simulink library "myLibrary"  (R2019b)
settings: Solver=VariableStepAuto  StartTime=0.0  StopTime=10.0  RelTol=1e-3
undefined symbols (not defined in the file or in its folder): batt_delay, Calculation, cap_1ph, cap_3ph, Complex, Current, Dynamic, EV, ev_charger, EV_ID, ev_num, gcbh, Iabc, Load, max_charge_1ph, max_charge_3ph, max_disch_1ph, max_disch_3ph, MV_LV_transf, myLibrary, phase, Phase, Phasor, rated_1ph, rated_3ph, Single, SoC_init, SPDL, sps_rtmsupport, Tr_capacity, Tstep, Vabc, Vnom, yes
libraries: powerlib x163, $bdroot x13, spsVIMeasurementModel x3, simulink x2, powerlib_meascontrol x1
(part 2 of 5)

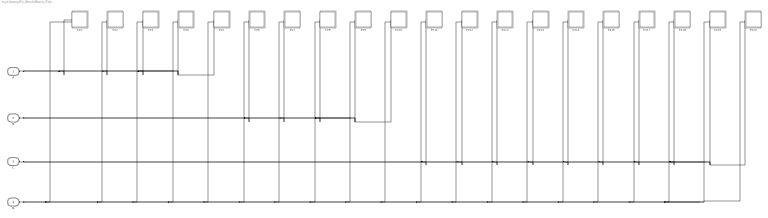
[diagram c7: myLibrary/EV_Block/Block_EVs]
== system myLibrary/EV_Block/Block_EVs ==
  EV1 : Subsystem  mask(Single-Phase Dynamic Load){Load_Profile=EV(1), Phase=1}
      mask prompts: Phase "Phase [A=1, B=2, C=3]"
      mask help: Single Phase Dynamic Load. The Load Profile is given by an external file.
  EV10 : Subsystem  mask(Single-Phase Dynamic Load){Load_Profile=EV(10), Phase=2}
      mask prompts: Phase "Phase [A=1, B=2, C=3]"
      mask help: Single Phase Dynamic Load. The Load Profile is given by an external file.
  EV11 : Subsystem  mask(Single-Phase Dynamic Load){Load_Profile=EV(11), Phase=3}
      mask prompts: Phase "Phase [A=1, B=2, C=3]"
      mask help: Single Phase Dynamic Load. The Load Profile is given by an external file.
  EV12 : Subsystem  mask(Single-Phase Dynamic Load){Load_Profile=EV(12), Phase=3}
      mask prompts: Phase "Phase [A=1, B=2, C=3]"
      mask help: Single Phase Dynamic Load. The Load Profile is given by an external file.
  EV13 : Subsystem  mask(Single-Phase Dynamic Load){Load_Profile=EV(13), Phase=3}
      mask prompts: Phase "Phase [A=1, B=2, C=3]"
      mask help: Single Phase Dynamic Load. The Load Profile is given by an external file.
  EV14 : Subsystem  mask(Single-Phase Dynamic Load){Load_Profile=EV(14), Phase=3}
      mask prompts: Phase "Phase [A=1, B=2, C=3]"
      mask help: Single Phase Dynamic Load. The Load Profile is given by an external file.
  EV15 : Subsystem  mask(Single-Phase Dynamic Load){Load_Profile=EV(15), Phase=3}
      mask prompts: Phase "Phase [A=1, B=2, C=3]"
      mask help: Single Phase Dynamic Load. The Load Profile is given by an external file.
  EV16 : Subsystem  mask(Single-Phase Dynamic Load){Load_Profile=EV(16), Phase=3}
      mask prompts: Phase "Phase [A=1, B=2, C=3]"
      mask help: Single Phase Dynamic Load. The Load Profile is given by an external file.
  EV17 : Subsystem  mask(Single-Phase Dynamic Load){Load_Profile=EV(17), Phase=3}
      mask prompts: Phase "Phase [A=1, B=2, C=3]"
      mask help: Single Phase Dynamic Load. The Load Profile is given by an external file.
  EV18 : Subsystem  mask(Single-Phase Dynamic Load){Load_Profile=EV(18), Phase=3}
      mask prompts: Phase "Phase [A=1, B=2, C=3]"
      mask help: Single Phase Dynamic Load. The Load Profile is given by an external file.
  EV19 : Subsystem  mask(Single-Phase Dynamic Load){Load_Profile=EV(19), Phase=3}
      mask prompts: Phase "Phase [A=1, B=2, C=3]"
      mask help: Single Phase Dynamic Load. The Load Profile is given by an external file.
  EV2 : Subsystem  mask(Single-Phase Dynamic Load){Load_Profile=EV(2), Phase=1}
      mask prompts: Phase "Phase [A=1, B=2, C=3]"
      mask help: Single Phase Dynamic Load. The Load Profile is given by an external file.
  EV20 : Subsystem  mask(Single-Phase Dynamic Load){Load_Profile=EV(20), Phase=3}
      mask prompts: Phase "Phase [A=1, B=2, C=3]"
      mask help: Single Phase Dynamic Load. The Load Profile is given by an external file.
  EV3 : Subsystem  mask(Single-Phase Dynamic Load){Load_Profile=EV(3), Phase=1}
      mask prompts: Phase "Phase [A=1, B=2, C=3]"
      mask help: Single Phase Dynamic Load. The Load Profile is given by an external file.
  EV4 : Subsystem  mask(Single-Phase Dynamic Load){Load_Profile=EV(4), Phase=1}
      mask prompts: Phase "Phase [A=1, B=2, C=3]"
      mask help: Single Phase Dynamic Load. The Load Profile is given by an external file.
  EV5 : Subsystem  mask(Single-Phase Dynamic Load){Load_Profile=EV(5), Phase=1}
      mask prompts: Phase "Phase [A=1, B=2, C=3]"
      mask help: Single Phase Dynamic Load. The Load Profile is given by an external file.
  EV6 : Subsystem  mask(Single-Phase Dynamic Load){Load_Profile=EV(6), Phase=2}
      mask prompts: Phase "Phase [A=1, B=2, C=3]"
      mask help: Single Phase Dynamic Load. The Load Profile is given by an external file.
  EV7 : Subsystem  mask(Single-Phase Dynamic Load){Load_Profile=EV(7), Phase=2}
      mask prompts: Phase "Phase [A=1, B=2, C=3]"
      mask help: Single Phase Dynamic Load. The Load Profile is given by an external file.
  EV8 : Subsystem  mask(Single-Phase Dynamic Load){Load_Profile=EV(8), Phase=2}
      mask prompts: Phase "Phase [A=1, B=2, C=3]"
      mask help: Single Phase Dynamic Load. The Load Profile is given by an external file.
  EV9 : Subsystem  mask(Single-Phase Dynamic Load){Load_Profile=EV(9), Phase=2}
      mask prompts: Phase "Phase [A=1, B=2, C=3]"
      mask help: Single Phase Dynamic Load. The Load Profile is given by an external file.
  A : PMIOPort  Tag=PMCPort  Side=Left
  B : PMIOPort  Tag=PMCPort  Port=2  Side=Left
  C : PMIOPort  Tag=PMCPort  Port=3  Side=Left
  N : PMIOPort  Tag=PMCPort  Port=4  Side=Left
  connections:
  N/RConn1 -- EV1/LConn2 -- EV2/LConn2 -- EV3/LConn2 -- EV4/LConn2 -- EV5/LConn2 -- EV6/LConn2 -- EV7/LConn2 -- EV8/LConn2 -- EV9/LConn2 -- EV10/LConn2 -- EV11/LConn2 -- EV12/LConn2 -- EV13/LConn2 -- EV14/LConn2 -- EV15/LConn2 -- EV16/LConn2 -- EV17/LConn2 -- EV18/LConn2 -- EV20/LConn2 -- EV19/LConn2
  A/RConn1 -- EV1/LConn1 -- EV2/LConn1 -- EV3/LConn1 -- EV5/LConn1 -- EV4/LConn1
  B/RConn1 -- EV6/LConn1 -- EV7/LConn1 -- EV8/LConn1 -- EV10/LConn1 -- EV9/LConn1
  C/RConn1 -- EV11/LConn1 -- EV12/LConn1 -- EV13/LConn1 -- EV14/LConn1 -- EV15/LConn1 -- EV16/LConn1 -- EV17/LConn1 -- EV18/LConn1 -- EV20/LConn1 -- EV19/LConn1

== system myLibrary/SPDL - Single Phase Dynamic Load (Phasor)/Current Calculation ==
  Vp : Inport
  Demux : Demux  Outputs=2
  Divide : Product  Inputs=*/
  From Workspace : FromWorkspace  VariableName=Load_Profile  SampleTime=0  OutputAfterFinalValue=Holding final value
  Gain : Gain  Gain=2
  Math Function : Math  Operator=conj
  Real-Imag to Complex : RealImagToComplex
  Isignal : Outport  VectorParamsAs1DForOutWhenUnconnected=off
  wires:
  From Workspace/1 -> Demux/1
  Real-Imag to Complex/1 -> Gain/1
  Vp/1 -> Divide/2
  Gain/1 -> Divide/1
  Divide/1 -> Math Function/1
  Math Function/1 -> Isignal/1
  Demux/1 -> Real-Imag to Complex/1
  Demux/2 -> Real-Imag to Complex/2

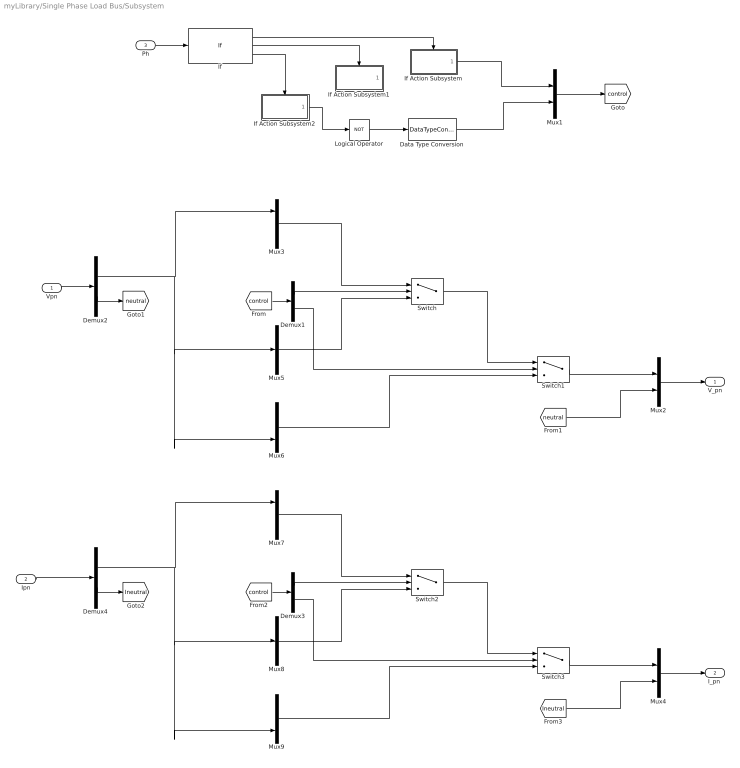
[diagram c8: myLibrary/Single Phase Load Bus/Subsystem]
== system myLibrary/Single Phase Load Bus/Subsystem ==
  Vpn : Inport
  Ipn : Inport  Port=2
  Ph : Inport  Port=3
  Data Type Conversion : DataTypeConversion  OutDataTypeStr=double
  Demux{1..4} (4 alike) : Demux  Outputs=2
  If : If  IfExpression=u1==1  ElseIfExpressions=u1==2
  If Action Subsystem : Subsystem  TreatAsAtomicUnit=on
  If Action Subsystem1 : Subsystem  TreatAsAtomicUnit=on
  If Action Subsystem2 : Subsystem  TreatAsAtomicUnit=on
  Logical Operator : Logic  Operator=NOT  AllPortsSameDT=off  OutDataTypeStr=boolean
  Mux1 : Mux  Inputs=2
  Mux2 : Mux  Inputs=2
  Mux{3,5..9} (6 alike) : Mux  Inputs=3
  Mux4 : Mux  Inputs=2
  Switch{,1..3} (4 alike) : Switch  Criteria=u2 > Threshold
  V_pn : Outport  VectorParamsAs1DForOutWhenUnconnected=off
  "I_pn " : Outport  Port=2  VectorParamsAs1DForOutWhenUnconnected=off
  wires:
  [control] -> Demux3/1
  Switch2/1 -> Switch3/1
  Demux4/2 -> [Ineutral]
  [Ineutral] -> Mux4/2
  Demux4/1 -> Mux7/1, Mux8/2, Mux9/3
  Mux4/1 -> "I_pn "/1
  Ipn/1 -> Demux4/1
  Mux9/1 -> Switch3/3
  Mux7/1 -> Switch2/1
  Mux8/1 -> Switch2/3
  Demux3/2 -> Switch3/2
  Switch3/1 -> Mux4/1
  Demux3/1 -> Switch2/2
  Mux2/1 -> V_pn/1
  [neutral] -> Mux2/2
  Demux2/2 -> [neutral]
  Switch1/1 -> Mux2/1
  Demux1/1 -> Switch/2
  Demux1/2 -> Switch1/2
  [control] -> Demux1/1
  Mux1/1 -> [control]
  Logical Operator/1 -> Data Type Conversion/1
  If Action Subsystem/1(Out1) -> Mux1/1
  If Action Subsystem2/1(Out1) -> Logical Operator/1
  If/3 -> If Action Subsystem2/Action
  If/2 -> If Action Subsystem1/Action
  If/1 -> If Action Subsystem/Action
  Ph/1 -> If/1
  Mux3/1 -> Switch/1
  Mux6/1 -> Switch1/3
  Switch/1 -> Switch1/1
  Demux2/1 -> Mux3/1, Mux5/2, Mux6/3
  Vpn/1 -> Demux2/1
  Mux5/1 -> Switch/3
  Data Type Conversion/1 -> Mux1/2

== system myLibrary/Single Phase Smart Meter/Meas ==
  Vpn : Inport
  Ipn : Inport  Port=2
  Vpg : Inport  Port=3
  Complex to Magnitude-Angle : ComplexToMagnitudeAngle
  Complex to Magnitude-Angle1 : ComplexToMagnitudeAngle
  Demux1 : Demux  Outputs=2
  Demux2 : Demux  Outputs=2
  Mag_To_RMS : Gain  Gain=1/sqrt(2)
  Mag_To_RMS1 : Gain  Gain=1/sqrt(2)
  Mux : Mux  Inputs=2
  Mux1 : Mux  Inputs=2
  Mux5 : Mux  Inputs=2
  PQ : Subsystem
  Measurements : Outport  VectorParamsAs1DForOutWhenUnconnected=off
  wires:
  Ipn/1 -> Demux1/1
  Mag_To_RMS1/1 -> Mux/2
  PQ/1(P) -> Mux1/1
  PQ/2(Q) -> Mux1/2
  Mux5/1 -> Measurements/1
  Mux/1 -> Mux5/2
  Mux1/1 -> Mux5/1
  Mag_To_RMS/1 -> Mux/1
  Demux1/1 -> PQ/2(I), Complex to Magnitude-Angle1/1
  Complex to Magnitude-Angle/1 -> Mag_To_RMS/1
  Complex to Magnitude-Angle1/1 -> Mag_To_RMS1/1
  Vpg/1 -> Demux2/1
  Vpn/1 -> PQ/1(V), Complex to Magnitude-Angle/1

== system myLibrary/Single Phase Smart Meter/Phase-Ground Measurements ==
  Current Measurement1 : powerlib/Measurements/Current Measurement  PhasorSimulation=off  OutputType=Complex  PSBequivalent=0
  Current Measurement4 : powerlib/Measurements/Current Measurement  PhasorSimulation=off  OutputType=Complex  PSBequivalent=0
  Ground1 : powerlib/Elements/Ground  LConnTagsString=a
  Ground2 : powerlib/Elements/Ground  LConnTagsString=a
  Mux : Mux  Inputs=2
  Mux1 : Mux  Inputs=2
  Voltage Measurement1 : powerlib/Measurements/Voltage Measurement  PhasorSimulation=off  OutputType=Complex  PSBequivalent=0
  Voltage Measurement3 : powerlib/Measurements/Voltage Measurement  PhasorSimulation=off  OutputType=Complex  PSBequivalent=0
  Phase : PMIOPort  Side=Left
  Neutral : PMIOPort  Port=2  Side=Left
  phase : PMIOPort  Port=3  Side=Right
  n : PMIOPort  Port=4  Side=Right
  Vp_Vn : Outport  VectorParamsAs1DForOutWhenUnconnected=off
  Ip_In : Outport  Port=2  VectorParamsAs1DForOutWhenUnconnected=off
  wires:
  Voltage Measurement1/1 -> Mux/1
  Voltage Measurement3/1 -> Mux/2
  Mux/1 -> Vp_Vn/1
  Current Measurement1/1 -> Mux1/1
  Current Measurement4/1 -> Mux1/2
  Mux1/1 -> Ip_In/1
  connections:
  Current Measurement1/RConn1 -- phase/RConn1
  Ground2/LConn1 -- Voltage Measurement1/LConn2
  Current Measurement4/LConn1 -- Neutral/RConn1 -- Voltage Measurement3/LConn1
  n/RConn1 -- Current Measurement4/RConn1
  Voltage Measurement3/LConn2 -- Ground1/LConn1
  Current Measurement1/LConn1 -- Phase/RConn1 -- Voltage Measurement1/LConn1

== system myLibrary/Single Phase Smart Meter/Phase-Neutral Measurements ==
  Voltage Measurement1 : powerlib/Measurements/Voltage Measurement  PhasorSimulation=off  OutputType=Complex  PSBequivalent=0
  Phase : PMIOPort  Side=Left
  Neutral : PMIOPort  Port=2  Side=Left
  Vpn : Outport  VectorParamsAs1DForOutWhenUnconnected=off
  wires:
  Voltage Measurement1/1 -> Vpn/1
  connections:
  Phase/RConn1 -- Voltage Measurement1/LConn1
  Neutral/RConn1 -- Voltage Measurement1/LConn2

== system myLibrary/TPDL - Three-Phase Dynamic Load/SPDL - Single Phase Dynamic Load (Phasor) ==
  Breaker : powerlib/Elements/Breaker  InitialState=1  SwitchingTimes=0  External=off  BreakerResistance=0.01  SnubberResistance=1e3  SnubberCapacitance=inf  Measurements=None  MoreParameters=on  NoBreakLoop=off
  Controlled Current Source : powerlib/Electrical Sources/Controlled Current Source  Initialize=on  Source_Type=AC  Amplitude=0  Phase=0  Frequency=50  Measurements=None
  Current Calculation : Subsystem
  Gain : Gain  Gain=sqrt(2)
  Snubber4 : powerlib/Elements/Series RLC Branch  LConnTagsString=__new0  RConnTagsString=__new0  BranchType=R  Resistance=1e6  Inductance=1e-3  SetiL0=off  InitialCurrent=0  Capacitance=1e-6  Setx0=off  InitialVoltage=0  Measurements=None
  Step : Step  Time=0.001  Before=-1  SampleTime=0
  Switch : Switch  Criteria=u2 > Threshold
  V Initialization : $bdroot/V Initialization  SystemSampleTime=-1  Latency=0  AutoFrameSizeCalculation=off
  Voltage Measurement : powerlib/Measurements/Voltage Measurement  PhasorSimulation=off  OutputType=Complex  PSBequivalent=0
  Phase : PMIOPort  Side=Left
  Neutral : PMIOPort  Port=2  Side=Left
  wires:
  Voltage Measurement/1 -> [Vm_c]
  Switch/1 -> Current Calculation/1(Vp)
  Current Calculation/1(Isignal) -> [Icontrol]
  [Icontrol] -> Controlled Current Source/1
  [Vm_c] -> Switch/1
  V Initialization/1 -> Gain/1
  Step/1 -> Switch/2
  Gain/1 -> Switch/3
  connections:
  Voltage Measurement/LConn1 -- Breaker/RConn1 -- Controlled Current Source/LConn1 -- Phase/RConn1
  Snubber4/RConn1 -- Controlled Current Source/RConn1 -- Voltage Measurement/LConn2 -- Neutral/RConn1
  Snubber4/LConn1 -- Breaker/LConn1

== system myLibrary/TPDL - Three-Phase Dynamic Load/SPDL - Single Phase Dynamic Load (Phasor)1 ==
  Breaker : powerlib/Elements/Breaker  InitialState=1  SwitchingTimes=0  External=off  BreakerResistance=0.01  SnubberResistance=1e3  SnubberCapacitance=inf  Measurements=None  MoreParameters=on  NoBreakLoop=off
  Controlled Current Source : powerlib/Electrical Sources/Controlled Current Source  Initialize=on  Source_Type=AC  Amplitude=0  Phase=0  Frequency=50  Measurements=None
  Current Calculation : Subsystem
  Gain : Gain  Gain=sqrt(2)
  Snubber4 : powerlib/Elements/Series RLC Branch  LConnTagsString=__new0  RConnTagsString=__new0  BranchType=R  Resistance=1e6  Inductance=1e-3  SetiL0=off  InitialCurrent=0  Capacitance=1e-6  Setx0=off  InitialVoltage=0  Measurements=None
  Step : Step  Time=0.001  Before=-1  SampleTime=0
  Switch : Switch  Criteria=u2 > Threshold
  V Initialization : $bdroot/V Initialization  SystemSampleTime=-1  Latency=0  AutoFrameSizeCalculation=off
  Voltage Measurement : powerlib/Measurements/Voltage Measurement  PhasorSimulation=off  OutputType=Complex  PSBequivalent=0
  Phase : PMIOPort  Side=Left
  Neutral : PMIOPort  Port=2  Side=Left
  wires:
  Voltage Measurement/1 -> [Vm_c]
  Switch/1 -> Current Calculation/1(Vp)
  Current Calculation/1(Isignal) -> [Icontrol]
  [Icontrol] -> Controlled Current Source/1
  [Vm_c] -> Switch/1
  Step/1 -> Switch/2
  Gain/1 -> Switch/3
  V Initialization/1 -> Gain/1
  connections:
  Breaker/LConn1 -- Snubber4/LConn1
  Snubber4/RConn1 -- Controlled Current Source/RConn1 -- Voltage Measurement/LConn2 -- Neutral/RConn1
  Breaker/RConn1 -- Voltage Measurement/LConn1 -- Phase/RConn1 -- Controlled Current Source/LConn1

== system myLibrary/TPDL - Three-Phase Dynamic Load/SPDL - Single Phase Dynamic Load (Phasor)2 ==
  Breaker : powerlib/Elements/Breaker  InitialState=1  SwitchingTimes=0  External=off  BreakerResistance=0.01  SnubberResistance=1e3  SnubberCapacitance=inf  Measurements=None  MoreParameters=on  NoBreakLoop=off
  Controlled Current Source : powerlib/Electrical Sources/Controlled Current Source  Initialize=on  Source_Type=AC  Amplitude=0  Phase=0  Frequency=50  Measurements=None
  Current Calculation : Subsystem
  Gain : Gain  Gain=sqrt(2)
  Snubber4 : powerlib/Elements/Series RLC Branch  LConnTagsString=__new0  RConnTagsString=__new0  BranchType=R  Resistance=1e6  Inductance=1e-3  SetiL0=off  InitialCurrent=0  Capacitance=1e-6  Setx0=off  InitialVoltage=0  Measurements=None
  Step : Step  Time=0.001  Before=-1  SampleTime=0
  Switch : Switch  Criteria=u2 > Threshold
  V Initialization : $bdroot/V Initialization  SystemSampleTime=-1  Latency=0  AutoFrameSizeCalculation=off
  Voltage Measurement : powerlib/Measurements/Voltage Measurement  PhasorSimulation=off  OutputType=Complex  PSBequivalent=0
  Phase : PMIOPort  Side=Left
  Neutral : PMIOPort  Port=2  Side=Left
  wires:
  Voltage Measurement/1 -> [Vm_c]
  Switch/1 -> Current Calculation/1(Vp)
  Current Calculation/1(Isignal) -> [Icontrol]
  [Icontrol] -> Controlled Current Source/1
  [Vm_c] -> Switch/1
  V Initialization/1 -> Gain/1
  Step/1 -> Switch/2
  Gain/1 -> Switch/3
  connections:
  Voltage Measurement/LConn1 -- Breaker/RConn1 -- Controlled Current Source/LConn1 -- Phase/RConn1
  Snubber4/RConn1 -- Controlled Current Source/RConn1 -- Voltage Measurement/LConn2 -- Neutral/RConn1
  Breaker/LConn1 -- Snubber4/LConn1

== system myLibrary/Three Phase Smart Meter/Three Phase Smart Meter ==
  Vabc : Inport
  Iabc : Inport  Port=2
  Complex to Magnitude-Angle : ComplexToMagnitudeAngle
  Complex to Magnitude-Angle1 : ComplexToMagnitudeAngle
  Demux : Demux  Outputs=3
  Demux1 : Demux  Outputs=3
  Mag_To_RMS : Gain  Gain=1/sqrt(2)
  Mag_To_RMS 2 : Gain  Gain=1/sqrt(2)
  Mux{,1..3,5} (5 alike) : Mux  Inputs=2
  Mux4 : Mux  Inputs=3
  PQ : Subsystem
  PQ 2 : Subsystem
  PQ 3 : Subsystem
  Meas. : Outport  VectorParamsAs1DForOutWhenUnconnected=off
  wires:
  PQ/1(P) -> Mux1/1
  PQ 3/1(P) -> Mux3/1
  PQ 2/1(P) -> Mux2/1
  PQ 2/2(Q) -> Mux2/2
  Mux1/1 -> Mux4/1
  Demux/3 -> PQ 3/1(V)
  Demux/1 -> PQ/1(V)
  PQ 3/2(Q) -> Mux3/2
  Demux1/3 -> PQ 3/2(I)
  Demux/2 -> PQ 2/1(V)
  Demux1/1 -> PQ/2(I)
  Demux1/2 -> PQ 2/2(I)
  Complex to Magnitude-Angle1/1 -> Mag_To_RMS 2/1
  Mux/1 -> Mux5/2
  Mux3/1 -> Mux4/3
  Complex to Magnitude-Angle/1 -> Mag_To_RMS/1
  Mag_To_RMS/1 -> Mux/1
  Vabc/1 -> Complex to Magnitude-Angle/1, Demux/1
  Mux5/1 -> Meas./1
  Mux2/1 -> Mux4/2
  Mux4/1 -> Mux5/1
  Mag_To_RMS 2/1 -> Mux/2
  Iabc/1 -> Complex to Magnitude-Angle1/1, Demux1/1
  PQ/2(Q) -> Mux1/2

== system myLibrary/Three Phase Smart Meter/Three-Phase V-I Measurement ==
  Kv : Gain  Gain=Ki
  Kv1 : Gain  Gain=Kv
  Mode I : spsVIMeasurementModel/Complex  SystemSampleTime=-1  Latency=0  AutoFrameSizeCalculation=off
  Mode V : spsVIMeasurementModel/Complex  SystemSampleTime=-1  Latency=0  AutoFrameSizeCalculation=off
  Model : spsVIMeasurementModel/VI  SystemSampleTime=-1  Latency=0  AutoFrameSizeCalculation=off
  A : PMIOPort  Side=Left
  B : PMIOPort  Port=2  Side=Left
  C : PMIOPort  Port=3  Side=Left
  a : PMIOPort  Port=4  Side=Right
  b : PMIOPort  Port=5  Side=Right
  c : PMIOPort  Port=6  Side=Right
  Vabc : Outport  VectorParamsAs1DForOutWhenUnconnected=off
  Iabc : Outport  Port=2  VectorParamsAs1DForOutWhenUnconnected=off
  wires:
  Model/2 -> Kv/1
  Model/1 -> Kv1/1
  Kv/1 -> Mode I/1
  Kv1/1 -> Mode V/1
  Mode I/1 -> Iabc/1
  Mode V/1 -> Vabc/1
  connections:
  Model/RConn3 -- c/RConn1
  Model/RConn1 -- a/RConn1
  Model/RConn2 -- b/RConn1
  Model/LConn3 -- C/RConn1
  Model/LConn1 -- A/RConn1
  Model/LConn2 -- B/RConn1

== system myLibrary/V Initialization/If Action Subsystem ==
  Action Port : ActionPort
  Constant : Constant
  Out1 : Outport  VectorParamsAs1DForOutWhenUnconnected=off
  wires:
  Constant/1 -> Out1/1

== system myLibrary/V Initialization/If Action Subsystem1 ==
  Action Port : ActionPort
  Constant : Constant
  Out1 : Outport  VectorParamsAs1DForOutWhenUnconnected=off
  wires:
  Constant/1 -> Out1/1

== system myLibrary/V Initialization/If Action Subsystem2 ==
  Action Port : ActionPort
  Constant : Constant
  Out1 : Outport  VectorParamsAs1DForOutWhenUnconnected=off
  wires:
  Constant/1 -> Out1/1

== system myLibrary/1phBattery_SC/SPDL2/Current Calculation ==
  Vp : Inport
  P : Inport  Port=2
  Q : Inport  Port=3
  Divide : Product  Inputs=*/
  Gain : Gain  Gain=2
  Math Function : Math  Operator=conj
  Real-Imag to Complex : RealImagToComplex
  Isignal : Outport  VectorParamsAs1DForOutWhenUnconnected=off
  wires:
  Real-Imag to Complex/1 -> Gain/1
  Vp/1 -> Divide/2
  Gain/1 -> Divide/1
  Divide/1 -> Math Function/1
  Math Function/1 -> Isignal/1
  P/1 -> Real-Imag to Complex/1
  Q/1 -> Real-Imag to Complex/2

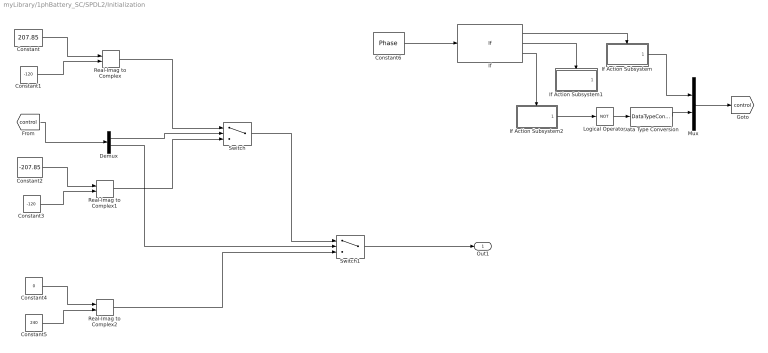
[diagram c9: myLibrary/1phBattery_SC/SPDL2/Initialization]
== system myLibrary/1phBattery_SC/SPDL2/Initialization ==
  Constant : Constant  Value=207.85
  Constant1 : Constant  Value=-120
  Constant2 : Constant  Value=-207.85
  Constant3 : Constant  Value=-120
  Constant4 : Constant  Value=0
  Constant5 : Constant  Value=240
  Constant6 : Constant  Value=Phase
  Data Type Conversion : DataTypeConversion  OutDataTypeStr=double
  Demux : Demux  Outputs=2
  If : If  IfExpression=u1 == 1  ElseIfExpressions=u1 == 2
  If Action Subsystem : Subsystem  TreatAsAtomicUnit=on
  If Action Subsystem1 : Subsystem  TreatAsAtomicUnit=on
  If Action Subsystem2 : Subsystem  TreatAsAtomicUnit=on
  Logical Operator : Logic  Operator=NOT  AllPortsSameDT=off  OutDataTypeStr=boolean
  Mux : Mux  Inputs=2
  Real-Imag to Complex : RealImagToComplex
  Real-Imag to Complex1 : RealImagToComplex
  Real-Imag to Complex2 : RealImagToComplex
  Switch : Switch  Criteria=u2 > Threshold
  Switch1 : Switch  Criteria=u2 > Threshold
  Out1 : Outport  VectorParamsAs1DForOutWhenUnconnected=off
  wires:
  Constant1/1 -> Real-Imag to Complex/2
  Constant/1 -> Real-Imag to Complex/1
  Constant3/1 -> Real-Imag to Complex1/2
  Constant2/1 -> Real-Imag to Complex1/1
  Constant5/1 -> Real-Imag to Complex2/2
  Constant4/1 -> Real-Imag to Complex2/1
  Real-Imag to Complex/1 -> Switch/1
  Real-Imag to Complex1/1 -> Switch/3
  Switch/1 -> Switch1/1
  Real-Imag to Complex2/1 -> Switch1/3
  Switch1/1 -> Out1/1
  Constant6/1 -> If/1
  If/1 -> If Action Subsystem/Action
  If/2 -> If Action Subsystem1/Action
  If/3 -> If Action Subsystem2/Action
  Demux/1 -> Switch/2
  Demux/2 -> Switch1/2
  If Action Subsystem2/1(Out1) -> Logical Operator/1
  Mux/1 -> [control]
  If Action Subsystem/1(Out1) -> Mux/1
  Logical Operator/1 -> Data Type Conversion/1
  [control] -> Demux/1
  Data Type Conversion/1 -> Mux/2

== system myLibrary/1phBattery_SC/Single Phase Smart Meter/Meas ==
  Vpn : Inport
  Ipn : Inport  Port=2
  Demux1 : Demux  Outputs=2
  PQ : Subsystem
  P : Outport  VectorParamsAs1DForOutWhenUnconnected=off
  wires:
  Vpn/1 -> PQ/1(V)
  Demux1/1 -> PQ/2(I)
  PQ/1(P) -> P/1
  Ipn/1 -> Demux1/1

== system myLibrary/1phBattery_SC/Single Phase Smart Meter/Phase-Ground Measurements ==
  Current Measurement1 : powerlib/Measurements/Current Measurement  PhasorSimulation=off  OutputType=Complex  PSBequivalent=0
  Current Measurement4 : powerlib/Measurements/Current Measurement  PhasorSimulation=off  OutputType=Complex  PSBequivalent=0
  Ground1 : powerlib/Elements/Ground  LConnTagsString=a
  Ground2 : powerlib/Elements/Ground  LConnTagsString=a
  Mux : Mux  Inputs=2
  Mux1 : Mux  Inputs=2
  Voltage Measurement1 : powerlib/Measurements/Voltage Measurement  PhasorSimulation=off  OutputType=Complex  PSBequivalent=0
  Voltage Measurement3 : powerlib/Measurements/Voltage Measurement  PhasorSimulation=off  OutputType=Complex  PSBequivalent=0
  Phase : PMIOPort  Side=Left
  Neutral : PMIOPort  Port=2  Side=Left
  phase : PMIOPort  Port=3  Side=Right
  n : PMIOPort  Port=4  Side=Right
  Vp_Vn : Outport  VectorParamsAs1DForOutWhenUnconnected=off
  Ip_In : Outport  Port=2  VectorParamsAs1DForOutWhenUnconnected=off
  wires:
  Mux1/1 -> Ip_In/1
  Current Measurement4/1 -> Mux1/2
  Current Measurement1/1 -> Mux1/1
  Mux/1 -> Vp_Vn/1
  Voltage Measurement3/1 -> Mux/2
  Voltage Measurement1/1 -> Mux/1
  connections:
  Voltage Measurement1/LConn1 -- Phase/RConn1 -- Current Measurement1/LConn1
  Voltage Measurement3/LConn2 -- Ground1/LConn1
  n/RConn1 -- Current Measurement4/RConn1
  Voltage Measurement3/LConn1 -- Neutral/RConn1 -- Current Measurement4/LConn1
  Ground2/LConn1 -- Voltage Measurement1/LConn2
  Current Measurement1/RConn1 -- phase/RConn1

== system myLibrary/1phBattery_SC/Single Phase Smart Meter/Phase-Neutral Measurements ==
  Voltage Measurement1 : powerlib/Measurements/Voltage Measurement  PhasorSimulation=off  OutputType=Complex  PSBequivalent=0
  Phase : PMIOPort  Side=Left
  Neutral : PMIOPort  Port=2  Side=Left
  Vpn : Outport  VectorParamsAs1DForOutWhenUnconnected=off
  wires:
  Voltage Measurement1/1 -> Vpn/1
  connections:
  Neutral/RConn1 -- Voltage Measurement1/LConn2
  Phase/RConn1 -- Voltage Measurement1/LConn1

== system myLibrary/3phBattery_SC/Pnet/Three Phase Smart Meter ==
  Vabc : Inport
  Iabc : Inport  Port=2
  Demux : Demux  Outputs=3
  Demux1 : Demux  Outputs=3
  PQ : Subsystem
  PQ 2 : Subsystem
  PQ 3 : Subsystem
  Sum : Sum  Inputs=3
  Sum1 : Sum  Inputs=3
  Pnet : Outport  VectorParamsAs1DForOutWhenUnconnected=off
  Qnet : Outport  Port=2  VectorParamsAs1DForOutWhenUnconnected=off
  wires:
  Sum1/1 -> Qnet/1
  PQ 3/2(Q) -> Sum1/3
  PQ 2/2(Q) -> Sum1/2
  PQ/2(Q) -> Sum1/1
  Sum/1 -> Pnet/1
  PQ/1(P) -> Sum/1
  Demux/3 -> PQ 3/1(V)
  Demux/1 -> PQ/1(V)
  Demux1/3 -> PQ 3/2(I)
  Demux/2 -> PQ 2/1(V)
  Demux1/1 -> PQ/2(I)
  Demux1/2 -> PQ 2/2(I)
  PQ 3/1(P) -> Sum/3
  Vabc/1 -> Demux/1
  PQ 2/1(P) -> Sum/2
  Iabc/1 -> Demux1/1

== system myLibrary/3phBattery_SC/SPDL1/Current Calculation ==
  Vp : Inport
  P : Inport  Port=2
  Q : Inport  Port=3
  Divide : Product  Inputs=*/
  Gain : Gain  Gain=2
  Math Function : Math  Operator=conj
  Real-Imag to Complex : RealImagToComplex
  Isignal : Outport  VectorParamsAs1DForOutWhenUnconnected=off
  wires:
  Real-Imag to Complex/1 -> Gain/1
  Vp/1 -> Divide/2
  Gain/1 -> Divide/1
  Divide/1 -> Math Function/1
  Math Function/1 -> Isignal/1
  P/1 -> Real-Imag to Complex/1
  Q/1 -> Real-Imag to Complex/2

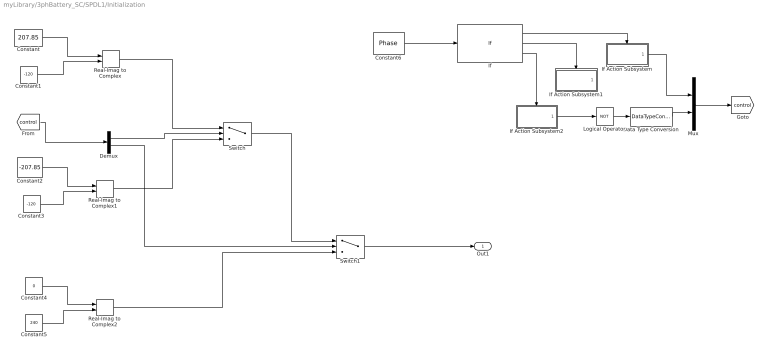
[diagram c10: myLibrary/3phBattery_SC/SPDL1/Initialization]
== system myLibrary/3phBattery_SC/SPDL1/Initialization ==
  Constant : Constant  Value=207.85
  Constant1 : Constant  Value=-120
  Constant2 : Constant  Value=-207.85
  Constant3 : Constant  Value=-120
  Constant4 : Constant  Value=0
  Constant5 : Constant  Value=240
  Constant6 : Constant  Value=Phase
  Data Type Conversion : DataTypeConversion  OutDataTypeStr=double
  Demux : Demux  Outputs=2
  If : If  IfExpression=u1 == 1  ElseIfExpressions=u1 == 2
  If Action Subsystem : Subsystem  TreatAsAtomicUnit=on
  If Action Subsystem1 : Subsystem  TreatAsAtomicUnit=on
  If Action Subsystem2 : Subsystem  TreatAsAtomicUnit=on
  Logical Operator : Logic  Operator=NOT  AllPortsSameDT=off  OutDataTypeStr=boolean
  Mux : Mux  Inputs=2
  Real-Imag to Complex : RealImagToComplex
  Real-Imag to Complex1 : RealImagToComplex
  Real-Imag to Complex2 : RealImagToComplex
  Switch : Switch  Criteria=u2 > Threshold
  Switch1 : Switch  Criteria=u2 > Threshold
  Out1 : Outport  VectorParamsAs1DForOutWhenUnconnected=off
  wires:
  Constant1/1 -> Real-Imag to Complex/2
  Constant/1 -> Real-Imag to Complex/1
  Constant3/1 -> Real-Imag to Complex1/2
  Constant2/1 -> Real-Imag to Complex1/1
  Constant5/1 -> Real-Imag to Complex2/2
  Constant4/1 -> Real-Imag to Complex2/1
  Real-Imag to Complex/1 -> Switch/1
  Real-Imag to Complex1/1 -> Switch/3
  Switch/1 -> Switch1/1
  Real-Imag to Complex2/1 -> Switch1/3
  Switch1/1 -> Out1/1
  Constant6/1 -> If/1
  If/1 -> If Action Subsystem/Action
  If/2 -> If Action Subsystem1/Action
  If/3 -> If Action Subsystem2/Action
  Demux/1 -> Switch/2
  Demux/2 -> Switch1/2
  If Action Subsystem2/1(Out1) -> Logical Operator/1
  Mux/1 -> [control]
  If Action Subsystem/1(Out1) -> Mux/1
  Logical Operator/1 -> Data Type Conversion/1
  [control] -> Demux/1
  Data Type Conversion/1 -> Mux/2

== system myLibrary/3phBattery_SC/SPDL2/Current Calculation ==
  Vp : Inport
  P : Inport  Port=2
  Q : Inport  Port=3
  Divide : Product  Inputs=*/
  Gain : Gain  Gain=2
  Math Function : Math  Operator=conj
  Real-Imag to Complex : RealImagToComplex
  Isignal : Outport  VectorParamsAs1DForOutWhenUnconnected=off
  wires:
  Real-Imag to Complex/1 -> Gain/1
  Vp/1 -> Divide/2
  Gain/1 -> Divide/1
  Divide/1 -> Math Function/1
  Math Function/1 -> Isignal/1
  P/1 -> Real-Imag to Complex/1
  Q/1 -> Real-Imag to Complex/2

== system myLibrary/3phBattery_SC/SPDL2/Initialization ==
  Constant : Constant  Value=207.85
  Constant1 : Constant  Value=-120
  Constant2 : Constant  Value=-207.85
  Constant3 : Constant  Value=-120
  Constant4 : Constant  Value=0
  Constant5 : Constant  Value=240
  Constant6 : Constant  Value=Phase
  Data Type Conversion : DataTypeConversion  OutDataTypeStr=double
  Demux : Demux  Outputs=2
  If : If  IfExpression=u1 == 1  ElseIfExpressions=u1 == 2
  If Action Subsystem : Subsystem  TreatAsAtomicUnit=on
  If Action Subsystem1 : Subsystem  TreatAsAtomicUnit=on
  If Action Subsystem2 : Subsystem  TreatAsAtomicUnit=on
  Logical Operator : Logic  Operator=NOT  AllPortsSameDT=off  OutDataTypeStr=boolean
  Mux : Mux  Inputs=2
  Real-Imag to Complex : RealImagToComplex
  Real-Imag to Complex1 : RealImagToComplex
  Real-Imag to Complex2 : RealImagToComplex
  Switch : Switch  Criteria=u2 > Threshold
  Switch1 : Switch  Criteria=u2 > Threshold
  Out1 : Outport  VectorParamsAs1DForOutWhenUnconnected=off
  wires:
  Constant1/1 -> Real-Imag to Complex/2
  Constant/1 -> Real-Imag to Complex/1
  Constant3/1 -> Real-Imag to Complex1/2
  Constant2/1 -> Real-Imag to Complex1/1
  Constant5/1 -> Real-Imag to Complex2/2
  Constant4/1 -> Real-Imag to Complex2/1
  Real-Imag to Complex/1 -> Switch/1
  Real-Imag to Complex1/1 -> Switch/3
  Switch/1 -> Switch1/1
  Real-Imag to Complex2/1 -> Switch1/3
  Switch1/1 -> Out1/1
  Constant6/1 -> If/1
  If/1 -> If Action Subsystem/Action
  If/2 -> If Action Subsystem1/Action
  If/3 -> If Action Subsystem2/Action
  Demux/1 -> Switch/2
  Demux/2 -> Switch1/2
  If Action Subsystem2/1(Out1) -> Logical Operator/1
  Mux/1 -> [control]
  If Action Subsystem/1(Out1) -> Mux/1
  Logical Operator/1 -> Data Type Conversion/1
  [control] -> Demux/1
  Data Type Conversion/1 -> Mux/2

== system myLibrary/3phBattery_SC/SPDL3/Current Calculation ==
  Vp : Inport
  P : Inport  Port=2
  Q : Inport  Port=3
  Divide : Product  Inputs=*/
  Gain : Gain  Gain=2
  Math Function : Math  Operator=conj
  Real-Imag to Complex : RealImagToComplex
  Isignal : Outport  VectorParamsAs1DForOutWhenUnconnected=off
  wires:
  Real-Imag to Complex/1 -> Gain/1
  Vp/1 -> Divide/2
  Gain/1 -> Divide/1
  Divide/1 -> Math Function/1
  Math Function/1 -> Isignal/1
  P/1 -> Real-Imag to Complex/1
  Q/1 -> Real-Imag to Complex/2

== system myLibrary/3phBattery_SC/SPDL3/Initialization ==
  Constant : Constant  Value=207.85
  Constant1 : Constant  Value=-120
  Constant2 : Constant  Value=-207.85
  Constant3 : Constant  Value=-120
  Constant4 : Constant  Value=0
  Constant5 : Constant  Value=240
  Constant6 : Constant  Value=Phase
  Data Type Conversion : DataTypeConversion  OutDataTypeStr=double
  Demux : Demux  Outputs=2
  If : If  IfExpression=u1 == 1  ElseIfExpressions=u1 == 2
  If Action Subsystem : Subsystem  TreatAsAtomicUnit=on
  If Action Subsystem1 : Subsystem  TreatAsAtomicUnit=on
  If Action Subsystem2 : Subsystem  TreatAsAtomicUnit=on
  Logical Operator : Logic  Operator=NOT  AllPortsSameDT=off  OutDataTypeStr=boolean
  Mux : Mux  Inputs=2
  Real-Imag to Complex : RealImagToComplex
  Real-Imag to Complex1 : RealImagToComplex
  Real-Imag to Complex2 : RealImagToComplex
  Switch : Switch  Criteria=u2 > Threshold
  Switch1 : Switch  Criteria=u2 > Threshold
  Out1 : Outport  VectorParamsAs1DForOutWhenUnconnected=off
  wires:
  Constant1/1 -> Real-Imag to Complex/2
  Constant/1 -> Real-Imag to Complex/1
  Constant3/1 -> Real-Imag to Complex1/2
  Constant2/1 -> Real-Imag to Complex1/1
  Constant5/1 -> Real-Imag to Complex2/2
  Constant4/1 -> Real-Imag to Complex2/1
  Real-Imag to Complex/1 -> Switch/1
  Real-Imag to Complex1/1 -> Switch/3
  Switch/1 -> Switch1/1
  Real-Imag to Complex2/1 -> Switch1/3
  Switch1/1 -> Out1/1
  Constant6/1 -> If/1
  If/1 -> If Action Subsystem/Action
  If/2 -> If Action Subsystem1/Action
  If/3 -> If Action Subsystem2/Action
  Demux/1 -> Switch/2
  Demux/2 -> Switch1/2
  If Action Subsystem2/1(Out1) -> Logical Operator/1
  Mux/1 -> [control]
  If Action Subsystem/1(Out1) -> Mux/1
  Logical Operator/1 -> Data Type Conversion/1
  [control] -> Demux/1
  Data Type Conversion/1 -> Mux/2

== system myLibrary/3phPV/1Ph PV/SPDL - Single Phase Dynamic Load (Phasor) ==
  Vm_c : Inport
  Breaker : powerlib/Elements/Breaker  InitialState=1  SwitchingTimes=0  External=off  BreakerResistance=0.01  SnubberResistance=1e3  SnubberCapacitance=inf  Measurements=None  MoreParameters=on  NoBreakLoop=off
  Controlled Current Source : powerlib/Electrical Sources/Controlled Current Source  Initialize=on  Source_Type=AC  Amplitude=0  Phase=0  Frequency=50  Measurements=None
  Current Calculation : Subsystem  AncestorBlock=myLibrary/SPDL - Single Phase Dynamic Load (Phasor)1/Current Calculation
  Gain : Gain  Gain=sqrt(2)
  Snubber4 : powerlib/Elements/Series RLC Branch  LConnTagsString=__new0  RConnTagsString=__new0  BranchType=R  Resistance=1e6  Inductance=1e-3  SetiL0=off  InitialCurrent=0  Capacitance=1e-6  Setx0=off  InitialVoltage=0  Measurements=None
  Step : Step  Time=0.001  Before=-1  SampleTime=0
  Switch : Switch  Criteria=u2 > Threshold
  V Initialization : $bdroot/V Initialization  SystemSampleTime=-1  Latency=0  AutoFrameSizeCalculation=off
  Phase : PMIOPort  Side=Left
  Neutral : PMIOPort  Port=2  Side=Left
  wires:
  Switch/1 -> Current Calculation/1(Vp)
  Current Calculation/1(Isignal) -> [Icontrol]
  [Icontrol] -> Controlled Current Source/1
  Vm_c/1 -> Switch/1
  V Initialization/1 -> Gain/1
  Step/1 -> Switch/2
  Gain/1 -> Switch/3
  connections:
  Neutral/RConn1 -- Snubber4/RConn1 -- Controlled Current Source/RConn1
  Controlled Current Source/LConn1 -- Breaker/RConn1 -- Phase/RConn1
  Snubber4/LConn1 -- Breaker/LConn1

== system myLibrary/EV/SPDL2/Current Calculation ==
  Vp : Inport
  P : Inport  Port=2
  Q : Inport  Port=3
  Divide : Product  Inputs=*/
  Gain : Gain  Gain=2
  Math Function : Math  Operator=conj
  Real-Imag to Complex : RealImagToComplex
  Isignal : Outport  VectorParamsAs1DForOutWhenUnconnected=off
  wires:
  Q/1 -> Real-Imag to Complex/2
  P/1 -> Real-Imag to Complex/1
  Math Function/1 -> Isignal/1
  Divide/1 -> Math Function/1
  Gain/1 -> Divide/1
  Vp/1 -> Divide/2
  Real-Imag to Complex/1 -> Gain/1

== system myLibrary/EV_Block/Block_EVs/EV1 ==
  Breaker : powerlib/Elements/Breaker  InitialState=1  SwitchingTimes=0  External=off  BreakerResistance=0.01  SnubberResistance=1e3  SnubberCapacitance=inf  Measurements=None  MoreParameters=on  NoBreakLoop=off
  Controlled Current Source : powerlib/Electrical Sources/Controlled Current Source  Initialize=on  Source_Type=AC  Amplitude=0  Phase=0  Frequency=50  Measurements=None
  Current Calculation : Subsystem
  Gain : Gain  Gain=sqrt(2)
  Initialization : Subsystem
  Snubber4 : powerlib/Elements/Series RLC Branch  LConnTagsString=__new0  RConnTagsString=__new0  BranchType=R  Resistance=1e6  Inductance=1e-3  SetiL0=off  InitialCurrent=0  Capacitance=1e-6  Setx0=off  InitialVoltage=0  Measurements=None
  Step : Step  Time=0.001  Before=-1  SampleTime=0
  Switch : Switch  Criteria=u2 > Threshold
  Voltage Measurement : powerlib/Measurements/Voltage Measurement  PhasorSimulation=off  OutputType=Complex  PSBequivalent=0
  Phase : PMIOPort  Side=Left
  Neutral : PMIOPort  Port=2  Side=Left
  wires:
  Gain/1 -> Switch/3
  Step/1 -> Switch/2
  Initialization/1(Out1) -> Gain/1
  [Vm_c] -> Switch/1
  [Icontrol] -> Controlled Current Source/1
  Current Calculation/1(Isignal) -> [Icontrol]
  Switch/1 -> Current Calculation/1(Vp)
  Voltage Measurement/1 -> [Vm_c]
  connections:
  Snubber4/LConn1 -- Breaker/LConn1
  Phase/RConn1 -- Voltage Measurement/LConn1 -- Breaker/RConn1 -- Controlled Current Source/LConn1
  Neutral/RConn1 -- Controlled Current Source/RConn1 -- Snubber4/RConn1 -- Voltage Measurement/LConn2

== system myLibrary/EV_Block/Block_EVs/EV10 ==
  Breaker : powerlib/Elements/Breaker  InitialState=1  SwitchingTimes=0  External=off  BreakerResistance=0.01  SnubberResistance=1e3  SnubberCapacitance=inf  Measurements=None  MoreParameters=on  NoBreakLoop=off
  Controlled Current Source : powerlib/Electrical Sources/Controlled Current Source  Initialize=on  Source_Type=AC  Amplitude=0  Phase=0  Frequency=50  Measurements=None
  Current Calculation : Subsystem
  Gain : Gain  Gain=sqrt(2)
  Initialization : Subsystem
  Snubber4 : powerlib/Elements/Series RLC Branch  LConnTagsString=__new0  RConnTagsString=__new0  BranchType=R  Resistance=1e6  Inductance=1e-3  SetiL0=off  InitialCurrent=0  Capacitance=1e-6  Setx0=off  InitialVoltage=0  Measurements=None
  Step : Step  Time=0.001  Before=-1  SampleTime=0
  Switch : Switch  Criteria=u2 > Threshold
  Voltage Measurement : powerlib/Measurements/Voltage Measurement  PhasorSimulation=off  OutputType=Complex  PSBequivalent=0
  Phase : PMIOPort  Side=Left
  Neutral : PMIOPort  Port=2  Side=Left
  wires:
  Gain/1 -> Switch/3
  Step/1 -> Switch/2
  Initialization/1(Out1) -> Gain/1
  [Vm_c] -> Switch/1
  [Icontrol] -> Controlled Current Source/1
  Current Calculation/1(Isignal) -> [Icontrol]
  Switch/1 -> Current Calculation/1(Vp)
  Voltage Measurement/1 -> [Vm_c]
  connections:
  Snubber4/LConn1 -- Breaker/LConn1
  Phase/RConn1 -- Voltage Measurement/LConn1 -- Breaker/RConn1 -- Controlled Current Source/LConn1
  Neutral/RConn1 -- Controlled Current Source/RConn1 -- Snubber4/RConn1 -- Voltage Measurement/LConn2

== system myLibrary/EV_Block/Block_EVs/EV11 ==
  Breaker : powerlib/Elements/Breaker  InitialState=1  SwitchingTimes=0  External=off  BreakerResistance=0.01  SnubberResistance=1e3  SnubberCapacitance=inf  Measurements=None  MoreParameters=on  NoBreakLoop=off
  Controlled Current Source : powerlib/Electrical Sources/Controlled Current Source  Initialize=on  Source_Type=AC  Amplitude=0  Phase=0  Frequency=50  Measurements=None
  Current Calculation : Subsystem
  Gain : Gain  Gain=sqrt(2)
  Initialization : Subsystem
  Snubber4 : powerlib/Elements/Series RLC Branch  LConnTagsString=__new0  RConnTagsString=__new0  BranchType=R  Resistance=1e6  Inductance=1e-3  SetiL0=off  InitialCurrent=0  Capacitance=1e-6  Setx0=off  InitialVoltage=0  Measurements=None
  Step : Step  Time=0.001  Before=-1  SampleTime=0
  Switch : Switch  Criteria=u2 > Threshold
  Voltage Measurement : powerlib/Measurements/Voltage Measurement  PhasorSimulation=off  OutputType=Complex  PSBequivalent=0
  Phase : PMIOPort  Side=Left
  Neutral : PMIOPort  Port=2  Side=Left
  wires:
  Gain/1 -> Switch/3
  Step/1 -> Switch/2
  Initialization/1(Out1) -> Gain/1
  [Vm_c] -> Switch/1
  [Icontrol] -> Controlled Current Source/1
  Current Calculation/1(Isignal) -> [Icontrol]
  Switch/1 -> Current Calculation/1(Vp)
  Voltage Measurement/1 -> [Vm_c]
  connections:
  Snubber4/LConn1 -- Breaker/LConn1
  Phase/RConn1 -- Voltage Measurement/LConn1 -- Breaker/RConn1 -- Controlled Current Source/LConn1
  Neutral/RConn1 -- Controlled Current Source/RConn1 -- Snubber4/RConn1 -- Voltage Measurement/LConn2

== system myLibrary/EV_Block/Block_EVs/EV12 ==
  Breaker : powerlib/Elements/Breaker  InitialState=1  SwitchingTimes=0  External=off  BreakerResistance=0.01  SnubberResistance=1e3  SnubberCapacitance=inf  Measurements=None  MoreParameters=on  NoBreakLoop=off
  Controlled Current Source : powerlib/Electrical Sources/Controlled Current Source  Initialize=on  Source_Type=AC  Amplitude=0  Phase=0  Frequency=50  Measurements=None
  Current Calculation : Subsystem
  Gain : Gain  Gain=sqrt(2)
  Initialization : Subsystem
  Snubber4 : powerlib/Elements/Series RLC Branch  LConnTagsString=__new0  RConnTagsString=__new0  BranchType=R  Resistance=1e6  Inductance=1e-3  SetiL0=off  InitialCurrent=0  Capacitance=1e-6  Setx0=off  InitialVoltage=0  Measurements=None
  Step : Step  Time=0.001  Before=-1  SampleTime=0
  Switch : Switch  Criteria=u2 > Threshold
  Voltage Measurement : powerlib/Measurements/Voltage Measurement  PhasorSimulation=off  OutputType=Complex  PSBequivalent=0
  Phase : PMIOPort  Side=Left
  Neutral : PMIOPort  Port=2  Side=Left
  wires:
  Gain/1 -> Switch/3
  Step/1 -> Switch/2
  Initialization/1(Out1) -> Gain/1
  [Vm_c] -> Switch/1
  [Icontrol] -> Controlled Current Source/1
  Current Calculation/1(Isignal) -> [Icontrol]
  Switch/1 -> Current Calculation/1(Vp)
  Voltage Measurement/1 -> [Vm_c]
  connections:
  Snubber4/LConn1 -- Breaker/LConn1
  Phase/RConn1 -- Voltage Measurement/LConn1 -- Breaker/RConn1 -- Controlled Current Source/LConn1
  Neutral/RConn1 -- Controlled Current Source/RConn1 -- Snubber4/RConn1 -- Voltage Measurement/LConn2

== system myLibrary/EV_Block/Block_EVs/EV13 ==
  Breaker : powerlib/Elements/Breaker  InitialState=1  SwitchingTimes=0  External=off  BreakerResistance=0.01  SnubberResistance=1e3  SnubberCapacitance=inf  Measurements=None  MoreParameters=on  NoBreakLoop=off
  Controlled Current Source : powerlib/Electrical Sources/Controlled Current Source  Initialize=on  Source_Type=AC  Amplitude=0  Phase=0  Frequency=50  Measurements=None
  Current Calculation : Subsystem
  Gain : Gain  Gain=sqrt(2)
  Initialization : Subsystem
  Snubber4 : powerlib/Elements/Series RLC Branch  LConnTagsString=__new0  RConnTagsString=__new0  BranchType=R  Resistance=1e6  Inductance=1e-3  SetiL0=off  InitialCurrent=0  Capacitance=1e-6  Setx0=off  InitialVoltage=0  Measurements=None
  Step : Step  Time=0.001  Before=-1  SampleTime=0
  Switch : Switch  Criteria=u2 > Threshold
  Voltage Measurement : powerlib/Measurements/Voltage Measurement  PhasorSimulation=off  OutputType=Complex  PSBequivalent=0
  Phase : PMIOPort  Side=Left
  Neutral : PMIOPort  Port=2  Side=Left
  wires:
  Gain/1 -> Switch/3
  Step/1 -> Switch/2
  Initialization/1(Out1) -> Gain/1
  [Vm_c] -> Switch/1
  [Icontrol] -> Controlled Current Source/1
  Current Calculation/1(Isignal) -> [Icontrol]
  Switch/1 -> Current Calculation/1(Vp)
  Voltage Measurement/1 -> [Vm_c]
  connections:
  Snubber4/LConn1 -- Breaker/LConn1
  Phase/RConn1 -- Voltage Measurement/LConn1 -- Breaker/RConn1 -- Controlled Current Source/LConn1
  Neutral/RConn1 -- Controlled Current Source/RConn1 -- Snubber4/RConn1 -- Voltage Measurement/LConn2

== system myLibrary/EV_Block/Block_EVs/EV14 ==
  Breaker : powerlib/Elements/Breaker  InitialState=1  SwitchingTimes=0  External=off  BreakerResistance=0.01  SnubberResistance=1e3  SnubberCapacitance=inf  Measurements=None  MoreParameters=on  NoBreakLoop=off
  Controlled Current Source : powerlib/Electrical Sources/Controlled Current Source  Initialize=on  Source_Type=AC  Amplitude=0  Phase=0  Frequency=50  Measurements=None
  Current Calculation : Subsystem
  Gain : Gain  Gain=sqrt(2)
  Initialization : Subsystem
  Snubber4 : powerlib/Elements/Series RLC Branch  LConnTagsString=__new0  RConnTagsString=__new0  BranchType=R  Resistance=1e6  Inductance=1e-3  SetiL0=off  InitialCurrent=0  Capacitance=1e-6  Setx0=off  InitialVoltage=0  Measurements=None
  Step : Step  Time=0.001  Before=-1  SampleTime=0
  Switch : Switch  Criteria=u2 > Threshold
  Voltage Measurement : powerlib/Measurements/Voltage Measurement  PhasorSimulation=off  OutputType=Complex  PSBequivalent=0
  Phase : PMIOPort  Side=Left
  Neutral : PMIOPort  Port=2  Side=Left
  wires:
  Gain/1 -> Switch/3
  Step/1 -> Switch/2
  Initialization/1(Out1) -> Gain/1
  [Vm_c] -> Switch/1
  [Icontrol] -> Controlled Current Source/1
  Current Calculation/1(Isignal) -> [Icontrol]
  Switch/1 -> Current Calculation/1(Vp)
  Voltage Measurement/1 -> [Vm_c]
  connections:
  Snubber4/LConn1 -- Breaker/LConn1
  Phase/RConn1 -- Voltage Measurement/LConn1 -- Breaker/RConn1 -- Controlled Current Source/LConn1
  Neutral/RConn1 -- Controlled Current Source/RConn1 -- Snubber4/RConn1 -- Voltage Measurement/LConn2

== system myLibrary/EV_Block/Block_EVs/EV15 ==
  Breaker : powerlib/Elements/Breaker  InitialState=1  SwitchingTimes=0  External=off  BreakerResistance=0.01  SnubberResistance=1e3  SnubberCapacitance=inf  Measurements=None  MoreParameters=on  NoBreakLoop=off
  Controlled Current Source : powerlib/Electrical Sources/Controlled Current Source  Initialize=on  Source_Type=AC  Amplitude=0  Phase=0  Frequency=50  Measurements=None
  Current Calculation : Subsystem
  Gain : Gain  Gain=sqrt(2)
  Initialization : Subsystem
  Snubber4 : powerlib/Elements/Series RLC Branch  LConnTagsString=__new0  RConnTagsString=__new0  BranchType=R  Resistance=1e6  Inductance=1e-3  SetiL0=off  InitialCurrent=0  Capacitance=1e-6  Setx0=off  InitialVoltage=0  Measurements=None
  Step : Step  Time=0.001  Before=-1  SampleTime=0
  Switch : Switch  Criteria=u2 > Threshold
  Voltage Measurement : powerlib/Measurements/Voltage Measurement  PhasorSimulation=off  OutputType=Complex  PSBequivalent=0
  Phase : PMIOPort  Side=Left
  Neutral : PMIOPort  Port=2  Side=Left
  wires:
  Gain/1 -> Switch/3
  Step/1 -> Switch/2
  Initialization/1(Out1) -> Gain/1
  [Vm_c] -> Switch/1
  [Icontrol] -> Controlled Current Source/1
  Current Calculation/1(Isignal) -> [Icontrol]
  Switch/1 -> Current Calculation/1(Vp)
  Voltage Measurement/1 -> [Vm_c]
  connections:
  Snubber4/LConn1 -- Breaker/LConn1
  Phase/RConn1 -- Voltage Measurement/LConn1 -- Breaker/RConn1 -- Controlled Current Source/LConn1
  Neutral/RConn1 -- Controlled Current Source/RConn1 -- Snubber4/RConn1 -- Voltage Measurement/LConn2

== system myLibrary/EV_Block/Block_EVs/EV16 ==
  Breaker : powerlib/Elements/Breaker  InitialState=1  SwitchingTimes=0  External=off  BreakerResistance=0.01  SnubberResistance=1e3  SnubberCapacitance=inf  Measurements=None  MoreParameters=on  NoBreakLoop=off
  Controlled Current Source : powerlib/Electrical Sources/Controlled Current Source  Initialize=on  Source_Type=AC  Amplitude=0  Phase=0  Frequency=50  Measurements=None
  Current Calculation : Subsystem
  Gain : Gain  Gain=sqrt(2)
  Initialization : Subsystem
  Snubber4 : powerlib/Elements/Series RLC Branch  LConnTagsString=__new0  RConnTagsString=__new0  BranchType=R  Resistance=1e6  Inductance=1e-3  SetiL0=off  InitialCurrent=0  Capacitance=1e-6  Setx0=off  InitialVoltage=0  Measurements=None
  Step : Step  Time=0.001  Before=-1  SampleTime=0
  Switch : Switch  Criteria=u2 > Threshold
  Voltage Measurement : powerlib/Measurements/Voltage Measurement  PhasorSimulation=off  OutputType=Complex  PSBequivalent=0
  Phase : PMIOPort  Side=Left
  Neutral : PMIOPort  Port=2  Side=Left
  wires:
  Gain/1 -> Switch/3
  Step/1 -> Switch/2
  Initialization/1(Out1) -> Gain/1
  [Vm_c] -> Switch/1
  [Icontrol] -> Controlled Current Source/1
  Current Calculation/1(Isignal) -> [Icontrol]
  Switch/1 -> Current Calculation/1(Vp)
  Voltage Measurement/1 -> [Vm_c]
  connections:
  Snubber4/LConn1 -- Breaker/LConn1
  Phase/RConn1 -- Voltage Measurement/LConn1 -- Breaker/RConn1 -- Controlled Current Source/LConn1
  Neutral/RConn1 -- Controlled Current Source/RConn1 -- Snubber4/RConn1 -- Voltage Measurement/LConn2

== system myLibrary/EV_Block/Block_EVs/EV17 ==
  Breaker : powerlib/Elements/Breaker  InitialState=1  SwitchingTimes=0  External=off  BreakerResistance=0.01  SnubberResistance=1e3  SnubberCapacitance=inf  Measurements=None  MoreParameters=on  NoBreakLoop=off
  Controlled Current Source : powerlib/Electrical Sources/Controlled Current Source  Initialize=on  Source_Type=AC  Amplitude=0  Phase=0  Frequency=50  Measurements=None
  Current Calculation : Subsystem
  Gain : Gain  Gain=sqrt(2)
  Initialization : Subsystem
  Snubber4 : powerlib/Elements/Series RLC Branch  LConnTagsString=__new0  RConnTagsString=__new0  BranchType=R  Resistance=1e6  Inductance=1e-3  SetiL0=off  InitialCurrent=0  Capacitance=1e-6  Setx0=off  InitialVoltage=0  Measurements=None
  Step : Step  Time=0.001  Before=-1  SampleTime=0
  Switch : Switch  Criteria=u2 > Threshold
  Voltage Measurement : powerlib/Measurements/Voltage Measurement  PhasorSimulation=off  OutputType=Complex  PSBequivalent=0
  Phase : PMIOPort  Side=Left
  Neutral : PMIOPort  Port=2  Side=Left
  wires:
  Gain/1 -> Switch/3
  Step/1 -> Switch/2
  Initialization/1(Out1) -> Gain/1
  [Vm_c] -> Switch/1
  [Icontrol] -> Controlled Current Source/1
  Current Calculation/1(Isignal) -> [Icontrol]
  Switch/1 -> Current Calculation/1(Vp)
  Voltage Measurement/1 -> [Vm_c]
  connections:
  Snubber4/LConn1 -- Breaker/LConn1
  Phase/RConn1 -- Voltage Measurement/LConn1 -- Breaker/RConn1 -- Controlled Current Source/LConn1
  Neutral/RConn1 -- Controlled Current Source/RConn1 -- Snubber4/RConn1 -- Voltage Measurement/LConn2

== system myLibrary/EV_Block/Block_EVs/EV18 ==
  Breaker : powerlib/Elements/Breaker  InitialState=1  SwitchingTimes=0  External=off  BreakerResistance=0.01  SnubberResistance=1e3  SnubberCapacitance=inf  Measurements=None  MoreParameters=on  NoBreakLoop=off
  Controlled Current Source : powerlib/Electrical Sources/Controlled Current Source  Initialize=on  Source_Type=AC  Amplitude=0  Phase=0  Frequency=50  Measurements=None
  Current Calculation : Subsystem
  Gain : Gain  Gain=sqrt(2)
  Initialization : Subsystem
  Snubber4 : powerlib/Elements/Series RLC Branch  LConnTagsString=__new0  RConnTagsString=__new0  BranchType=R  Resistance=1e6  Inductance=1e-3  SetiL0=off  InitialCurrent=0  Capacitance=1e-6  Setx0=off  InitialVoltage=0  Measurements=None
  Step : Step  Time=0.001  Before=-1  SampleTime=0
  Switch : Switch  Criteria=u2 > Threshold
  Voltage Measurement : powerlib/Measurements/Voltage Measurement  PhasorSimulation=off  OutputType=Complex  PSBequivalent=0
  Phase : PMIOPort  Side=Left
  Neutral : PMIOPort  Port=2  Side=Left
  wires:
  Gain/1 -> Switch/3
  Step/1 -> Switch/2
  Initialization/1(Out1) -> Gain/1
  [Vm_c] -> Switch/1
  [Icontrol] -> Controlled Current Source/1
  Current Calculation/1(Isignal) -> [Icontrol]
  Switch/1 -> Current Calculation/1(Vp)
  Voltage Measurement/1 -> [Vm_c]
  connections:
  Snubber4/LConn1 -- Breaker/LConn1
  Phase/RConn1 -- Voltage Measurement/LConn1 -- Breaker/RConn1 -- Controlled Current Source/LConn1
  Neutral/RConn1 -- Controlled Current Source/RConn1 -- Snubber4/RConn1 -- Voltage Measurement/LConn2
